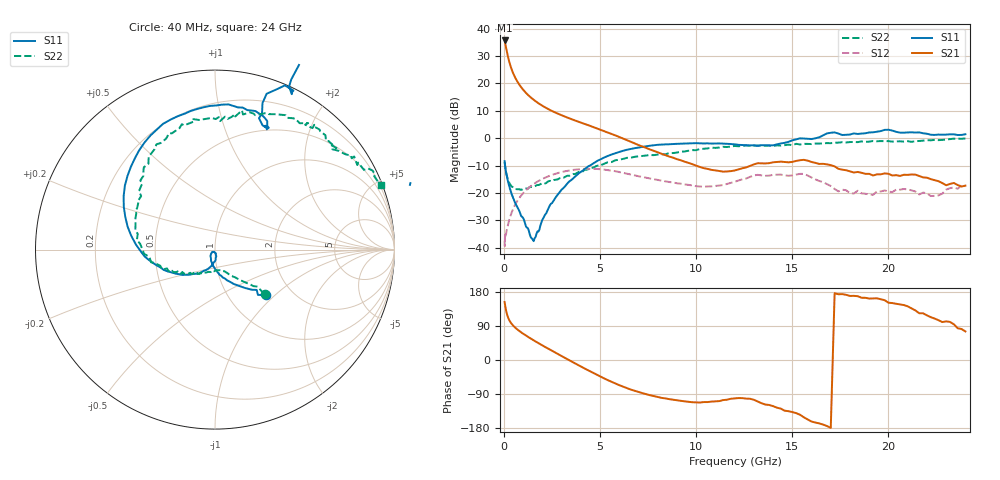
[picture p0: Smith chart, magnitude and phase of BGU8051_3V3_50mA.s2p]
! BGU8051_3V3_50mA
! Date/time Tue Jun 16 11:08:37 2015
! VAR V_out= 3.3000
! VAR I_out= 50.0000
! VAR V_in= 5.6400
! VAR I_in= 0.7041
# MHz S MA R 50
!  Freq-MHz  S11-mag  S11-arg  S21-mag  S21-arg  S12-mag  S12-arg  S22-mag  S22-arg
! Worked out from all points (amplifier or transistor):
!   187 points, 40 MHz to 24 GHz, reference 50 ohm
!   highest |S21| = 35.7 dB at 40 MHz (marker M1)
!   |S21| within 3 dB of that: start of sweep to 126.1 MHz
!   unconditionally stable (mu >= 1): 388.5 MHz to 13.05 GHz
!   at 750 MHz: K = 1.02, MAG = 20.5 dB, |S12| = -22.4 dB
!   at 5.4 GHz: K = 1.20, MAG = 4.2 dB, |S12| = -11.6 dB
!   at 24 GHz: K = 0.50, MSG = 0.1 dB, |S12| = -17.5 dB
!   lowest NFmin = 0.34 dB at 400 MHz
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40  0.382 -41.5  61.15 152.9  0.01338 30.9  0.3705 -41.7
60  0.3231 -44.0  56.99 146.6  0.01722 56.0  0.3143 -41.0
80  0.2914 -49.0  52.15 140.5  0.01565 39.9  0.2791 -44.5
120  0.2379 -57.2  44.36 129.7  0.0182 46.6  0.2324 -49.0
160  0.2005 -64.5  37.7 121.3  0.02165 50.6  0.2039 -52.5
200  0.1716 -70.7  32.42 114.8  0.02489 53.1  0.1819 -56.1
260  0.1418 -80.0  26.59 107.3  0.03017 57.6  0.1598 -59.8
320  0.1175 -85.4  22.35 101.7  0.03593 59.7  0.1448 -62.9
400  0.09578 -93.8  18.34 95.8  0.04296 61.5  0.1332 -66.1
500  0.07903 -100.0  14.95 89.9  0.05234 61.8  0.1245 -72.0
700  0.05529 -114.0  10.89 80.7  0.07146 60.3  0.1168 -79.1
900  0.03795 -127.9  8.556 73.0  0.08965 57.4  0.1144 -87.8
1150  0.02444 -136.5  6.74 64.5  0.1119 52.9  0.121 -97.6
1500  0.01415 -112.0  5.204 53.5  0.1416 45.7  0.1291 -106.5
2500  0.06503 -90.6  3.151 24.4  0.2133 23.3  0.1649 -127.2
4100  0.256 -148.3  1.88 -19.7  0.2742 -13.8  0.2468 -149.5
6000  0.561 154.9  1.052 -66.4  0.2412 -52.7  0.4045 179.8
8200  0.7659 108.7  0.5204 -100.0  0.168 -74.3  0.5073 147.9
12200  0.757 67.4  0.2692 -100.5  0.169 -73.6  0.7133 104.0
16200  0.9978 65.6  0.3548 -165.1  0.1771 -147.9  0.799 71.1
20200  1.379 31.8  0.2086 150.2  0.1034 -143.8  0.8663 44.5
24000  1.182 19.8  0.1362 75.4  0.1328 -162.4  0.9894 21.2
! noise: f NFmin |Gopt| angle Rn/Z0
400  0.3373  0.04873  107.1  0.0448
550  0.3464  0.05469  124.8  0.0457
950  0.3824  0.08023  153.4  0.0476
1250  0.4206  0.1015  165.7  0.0485
1600  0.4774  0.1258  176.2  0.0497
1900  0.5366  0.1462  183.6  0.051
2250  0.6179  0.1698  191.1  0.0534
2600  0.7123  0.1935  197.8  0.0571
3300  0.9405  0.2434  209.3  0.0705
4000  1.221  0.2976  218.4  0.0948
